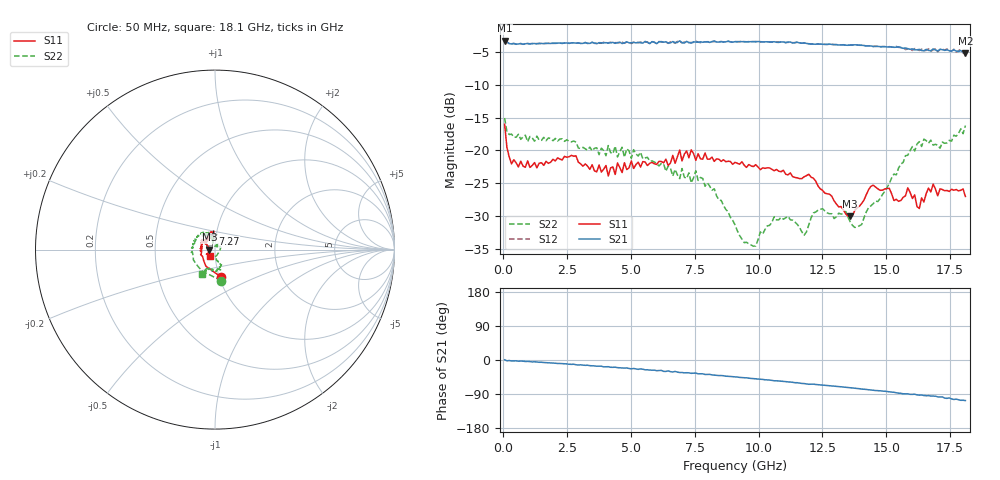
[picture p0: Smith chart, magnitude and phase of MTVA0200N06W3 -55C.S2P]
! Network Analyzer HP8720D.06.14 Serial No. US36140669
! 19 Aug 2005  14:30:02
! Frequency  S11  S21  S12  S22
# HZ  S  DB R 50
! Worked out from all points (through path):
!   201 points, 50 MHz to 18.1 GHz, reference 50 ohm
!   highest |S21| = -3.21 dB at 50 MHz (marker M1); lowest = -5.1 dB at 18.1 GHz (marker M2)
!   group delay of S21, straight-line fit = 16.3 ps
!   lowest |S11| = -30.1 dB at 13.59 GHz (marker M3), VSWR 1.06, Z = 47 - j0.0941 ohm
!   |S11| at or under -10 dB: start of sweep to end of sweep
!   |S22| runs from -34.6 to -15.0 dB; largest |S21 - S12| = 0.026
!   S11 on the Smith chart (normalised r, x): 50 MHz: 1.02, -0.32; 7.27 GHz: 0.96, +0.17; 18.1 GHz: 0.95, -0.07
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5e7  -15.99 -76.8  -3.21 0.5  -3.19 0.7  -15.04 -78.5
3.2075e8  -22.05 -150.9  -3.72 -2.6  -3.68 -2.5  -17.50 -154.9
2.66725e9  -20.74 144.3  -3.55 -11.5  -3.57 -11.7  -18.68 126.9
3.1185e9  -22.40 145.3  -3.63 -13.6  -3.65 -13.9  -19.52 130.4
4.11125e9  -23.90 128.6  -3.59 -17.7  -3.53 -18.7  -19.25 119.0
4.47225e9  -21.90 116.3  -3.52 -20.1  -3.53 -19.1  -20.99 121.0
6.09675e9  -21.67 103.7  -3.40 -27.9  -3.34 -27.8  -22.37 107.4
7.27e9  -21.12 98.6  -3.50 -33.8  -3.51 -35.1  -23.42 100.5
8.26275e9  -21.66 111.3  -3.26 -39.9  -3.36 -40.4  -25.84 100.7
9.075e9  -21.82 123.2  -3.37 -44.5  -3.36 -44.5  -31.36 107.4
9.88725e9  -22.17 126.0  -3.39 -49.6  -3.34 -49.6  -34.59 59.1
1.060925e10  -23.10 127.6  -3.38 -54.8  -3.45 -54.6  -30.12 41.0
1.17825e10  -24.02 149.0  -3.56 -62.2  -3.57 -62.3  -32.95 57.7
1.21435e10  -24.24 146.3  -3.75 -63.7  -3.72 -64.0  -29.54 67.4
1.35875e10  -30.08 -178.2  -3.90 -73.1  -3.86 -72.7  -30.89 0.0
1.403875e10  -28.08 -158.9  -3.92 -76.7  -3.93 -76.9  -31.31 -53.6
1.439975e10  -25.48 -151.9  -4.02 -79.1  -4.03 -79.0  -28.45 -86.9
1.512175e10  -25.79 -139.2  -4.18 -84.1  -4.13 -84.0  -25.02 -81.5
1.602425e10  -27.33 -120.1  -4.47 -90.7  -4.72 -90.9  -19.39 -69.2
1.6295e10  -28.87 -112.6  -4.55 -92.7  -4.72 -93.7  -18.64 -74.4
1.68365e10  -25.14 -130.9  -4.49 -95.4  -4.62 -97.0  -19.18 -98.7
1.81e10  -27.03 -126.9  -5.11 -107.0  -5.02 -107.8  -16.19 -118.0
